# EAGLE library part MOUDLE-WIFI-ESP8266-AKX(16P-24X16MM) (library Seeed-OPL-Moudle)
317060011
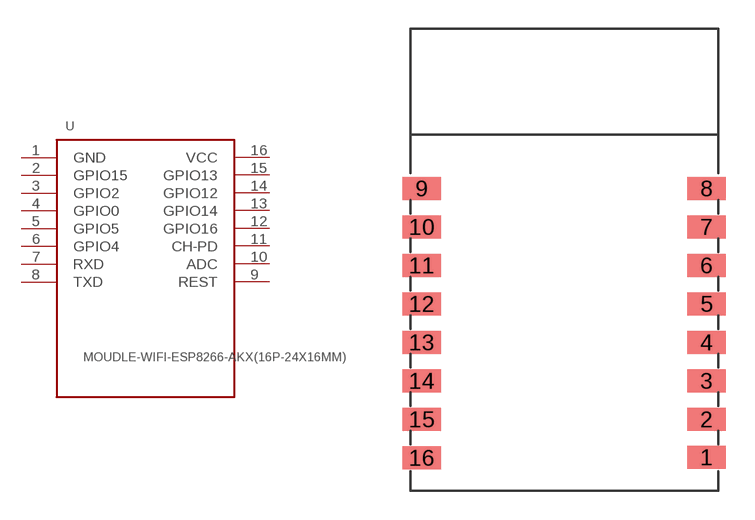
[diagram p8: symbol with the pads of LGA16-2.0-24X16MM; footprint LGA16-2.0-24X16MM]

Designator prefix U

## MOUDLE-WIFI-ESP8266-AKX(16P-24X16MM) (MPN: ES8266; VALUE: ES8266)  [LGA16-2.0-24X16MM]
1  GND
2  GPIO15
3  GPIO2
4  GPIO0
5  GPIO5
6  GPIO4
7  RXD
8  TXD
9  REST
10  ADC
11  CH-PD
12  GPIO16
13  GPIO14
14  GPIO12
15  GPIO13
16  VCC

## Footprint LGA16-2.0-24X16MM (pad centres in mm)
smd 2 x 1.2: 1 7.4,-10.27; 2 7.4,-8.3; 3 7.4,-6.3; 4 7.4,-4.3; 5 7.4,-2.3; 6 7.4,-0.3; 7 7.4,1.7; 8 7.4,3.7; 9 -7.4,3.7; 10 -7.4,1.7; 11 -7.4,-0.3; 12 -7.4,-2.3; 13 -7.4,-4.3; 14 -7.4,-6.3; 15 -7.4,-8.3; 16 -7.4,-10.3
